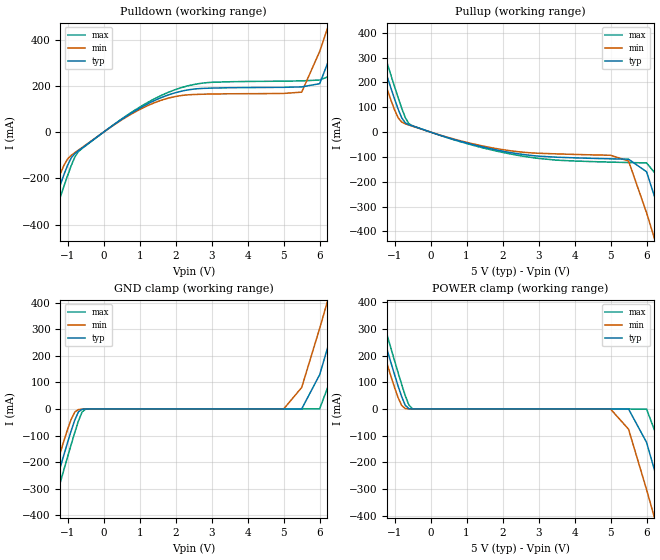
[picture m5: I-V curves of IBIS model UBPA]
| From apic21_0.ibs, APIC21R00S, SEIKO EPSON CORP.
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[Model]   UBPA
Model_type   I/O
Polarity   Non-Inverting
Vinh=2.0V
Vinl=0.8V
|   typ   min   max
C_comp   0   NA   NA
|   typ   min   max
[Voltage range]   5.0   4.5   5.5
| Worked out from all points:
|   slope of the pulldown table from 0 to 0.75 V, typ, clamps not added: 9.39 ohm
|   slope of the pullup table from 0 to 0.75 V, typ, clamps not added: 22.2 ohm
|   GND clamp passes 1 mA (typ) near -0.59 V on its own axis
|   POWER clamp passes 1 mA (typ) near -0.60 V on its own axis
[Pulldown]
|   Voltage   I(typ)   I(min)   I(max)
-10V      -4.572A    -4.493A    -4.652A
-1.9V     -557mA     -497.6mA   -617.7mA
-1.6V     -412.6mA   -355.8mA   -471.3mA
-1.1V     -182.7mA   -142.4mA   -232.8mA
-700mV    -80.49mA   -77.69mA   -84.24mA
1.5V      142.5mA    132.2mA    150.9mA
2.8V      189.1mA    163.9mA    212.6mA
5.5V      195.3mA    172.7mA    221.3mA
6V        209.2mA    348.3mA    225.1mA
6.5V      410.2mA    578.9mA    255.8mA
7V        644.6mA    815.5mA    474mA
10V       2.096A     2.262A     1.929A
[Pullup]
|   Voltage   I(typ)   I(min)   I(max)
-10V      4.473A     4.397A     4.549A
-1.8V     502mA      444.8mA    560.4mA
-1.6V     407.5mA    351.6mA    464.8mA
-1.5V     360.6mA    305.6mA    417.2mA
-900mV    92.72mA    57.98mA    138.8mA
-500mV    24.63mA    23.6mA     25.55mA
2.5V      -88.68mA   -80.06mA   -95.47mA
5.5V      -109.2mA   -116.4mA   -122.7mA
6V        -159.8mA   -324.7mA   -124.1mA
6.5V      -385.4mA   -562.4mA   -212.1mA
7V        -626.4mA   -804.7mA   -447.3mA
10V       -2.107A    -2.281A    -1.931A
[GND_clamp]
|   Voltage   I(typ)   I(min)   I(max)
-10V      -4.572A    -4.493A    -4.651A
-1.7V     -456.6mA   -397.1mA   -517.4mA
-1.5V     -360mA     -301.9mA   -419.6mA
-900mV    -81.25mA   -38.03mA   -132.6mA
-700mV    -10.92mA   -2.409mA   -45.16mA
-500mV    -160.3uA   -211.7uA   -494.9uA
5V        295.6pA    29.44uA    209.2pA
5.5V      39.62uA    80.6mA     278pA
6V        128.9mA    303mA      684.3uA
6.5V      358.9mA    537.3mA    181mA
7V        596mA      774.8mA    416.1mA
10V       2.043A     2.218A     1.867A
[POWER_clamp]
|   Voltage   I(typ)   I(min)   I(max)
-10V      4.473A     4.397A     4.549A
-1.7V     453.3mA    396.1mA    511.7mA
-1.5V     358.9mA    303mA      416.2mA
-900mV    85.64mA    42.21mA    135.4mA
-700mV    13.43mA    1.485mA    49.21mA
-500mV    39.62uA    29.44uA    685.5uA
5V        -494.5pA   -211.7uA   -408.1pA
5.5V      -160.3uA   -75.81mA   -478.4pA
6V        -125.1mA   -301.7mA   -494.8uA
6.5V      -359.9mA   -541.4mA   -179.1mA
7V        -602.6mA   -784.5mA   -419.6mA
10V       -2.084A    -2.262A    -1.905A
[Ramp]
|   V_typ   V_min   V_max
dV/dt_r   3.00/3.504e-10   2.70/3.642e-10   3.30/3.502e-10
dV/dt_f   3.00/3.299e-10   2.70/3.119e-10   3.30/3.022e-10
R_load = 5000ohm
